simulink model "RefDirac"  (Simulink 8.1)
settings: Solver=ode23t  StartTime=0.0  StopTime=tmax  RelTol=1e-3
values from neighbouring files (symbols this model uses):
  p = 66','Color','r')    [RefTrapecioModeladoM.m]    (also in RefTrapecioM.m = 66)
undefined symbols (not defined in the file or in its folder): k, ret

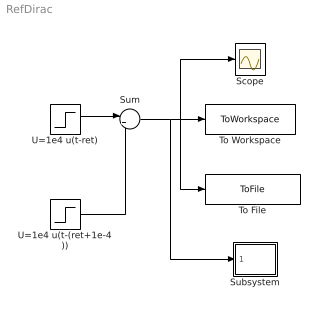
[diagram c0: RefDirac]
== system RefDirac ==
  Scope : Scope
  Subsystem : Subsystem
  Sum : Sum  Inputs=|+-
  To File : ToFile  Filename=Dirac.mat
  To Workspace : ToWorkspace  VariableName=Dirac  SampleTime=-1
  U=1e4 u(t-(ret+1e-4)) : Step  Time=ret+1e-4  After=1e4  SampleTime=0  ZeroCross=off
  U=1e4 u(t-ret) : Step  Time=ret  After=1e4  SampleTime=0  ZeroCross=off
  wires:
  U=1e4 u(t-(ret+1e-4))/1 -> Sum/2
  U=1e4 u(t-ret)/1 -> Sum/1
  Sum/1 -> Subsystem/1(Dirac), To File/1, To Workspace/1, Scope/1

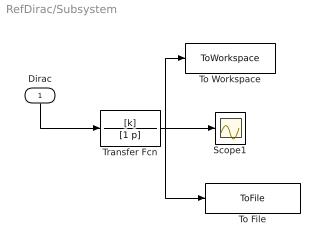
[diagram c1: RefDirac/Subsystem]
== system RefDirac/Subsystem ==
  Dirac : Inport
  Scope1 : Scope
  To File : ToFile  Filename=Impulso.mat
  To Workspace : ToWorkspace  VariableName=Impulso  SampleTime=-1
  Transfer Fcn : TransferFcn  Numerator=[k]  Denominator=[1 p]
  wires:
  Dirac/1 -> Transfer Fcn/1
  Transfer Fcn/1 -> To File/1, To Workspace/1, Scope1/1
